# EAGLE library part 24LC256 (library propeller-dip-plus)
256 Kbit (32 KByte) Industrial I2C Serial EEPROM
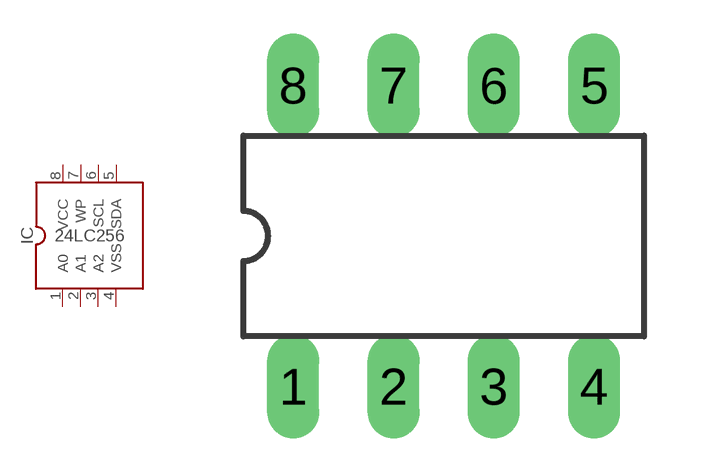
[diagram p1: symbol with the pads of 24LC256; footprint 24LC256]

Designator prefix IC

## 24LC256DIP-8  [24LC256]
1  A0  in
2  A1  in
3  A2  in
4  VSS  pwr
5  SDA
6  SCL  in
7  WP  in
8  VCC  pwr

## Footprint 24LC256 (pad centres in mm)
256 Kbit (32 KByte) Industrial I2C Serial EEPROM
drill 0.813 long: 1 -3.81,-3.81; 2 -1.27,-3.81; 3 1.27,-3.81; 4 3.81,-3.81; 5 3.81,3.81; 6 1.27,3.81; 7 -1.27,3.81; 8 -3.81,3.81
